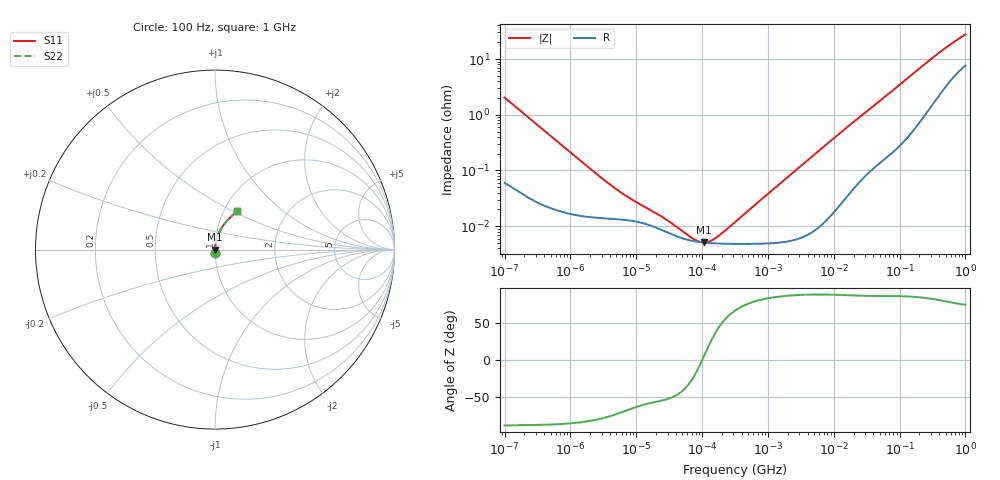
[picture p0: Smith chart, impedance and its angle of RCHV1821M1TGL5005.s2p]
! RCHV1821M1TGL5005  S-PARAMETER MODEL  (AEC-Q200 qualified)
! Model Generated by ELNA Corporation (http://www.ty-top.com)
! Version 1.0
! ELNA Control No. 240229
! Copyright (c) 2024 ELNA CO.,LTD. All Rights Reserved.
! Products Name : CONDUCTIVE POLYMER HYBRID ALUMINUM ELECTROLYTIC CAPACITORS
! Characteristics :
!  Capacitance  :  820uF  ,  Rated voltage  :  25V
!  Operating Temp. Range  :  -55 to +105 degC  ,  Endurance  :  5000hr at 105 degC
!  Dimension D  :  12.5mm  ,  Dimension L  :  13.5mm
! Frequency Range : 100Hz - 1GHz
! External Node Assignments :
!  1  o---| |---o  2
# MHz S RI R 50
!Freq[MHz].  S11 Real  S11 Imag  S21 Real  S21 Imag  S12 Real  S12 Imag  S22 Real  S22 Imag
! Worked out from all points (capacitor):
!   401 points, 100 Hz to 1 GHz, reference 50 ohm
!   read as one part in series: C = 781 uF near 108 Hz
!   lowest |Z| = 5.11 mohm at 106.5 kHz (marker M1)
!   series resonance near 101.1 kHz, so ESL is about 3.2 nH
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0.0001  0.00101 -0.0202  0.999 0.0202  0.999 0.0202  0.00101 -0.0202
0.000133  0.000726 -0.0153  0.9993 0.0153  0.9993 0.0153  0.000726 -0.0153
0.001488  0.000154 -0.00142  0.9998 0.00142  0.9998 0.00142  0.000154 -0.00142
0.00333  0.000139 -0.000645  0.9999 0.000645  0.9999 0.000645  0.000139 -0.000645
0.005855  0.000132 -0.000381  0.9999 0.000381  0.9999 0.000381  0.000132 -0.000381
0.00912  0.000123 -0.000261  0.9999 0.000261  0.9999 0.000261  0.000123 -0.000261
0.022131  8.97e-05 -0.000132  0.9999 0.000132  0.9999 0.000132  8.97e-05 -0.000132
0.037368  6.88e-05 -8.02e-05  0.9999 8.02e-05  0.9999 8.02e-05  6.88e-05 -8.02e-05
0.040504  6.63e-05 -7.3e-05  0.9999 7.3e-05  0.9999 7.3e-05  6.63e-05 -7.3e-05
0.043904  6.41e-05 -6.59e-05  0.9999 6.59e-05  0.9999 6.59e-05  6.41e-05 -6.59e-05
0.106537  5.1e-05 4e-06  0.9999 -4e-06  0.9999 -4e-06  5.1e-05 4e-06
0.248313  4.84e-05 7.88e-05  1 -7.88e-05  1 -7.88e-05  4.84e-05 7.88e-05
0.280221  4.83e-05 9.27e-05  1 -9.27e-05  1 -9.27e-05  4.83e-05 9.27e-05
0.316228  4.82e-05 0.000108  1 -0.000108  1 -0.000108  4.82e-05 0.000108
4.704354  8.12e-05 0.00179  0.9999 -0.00179  0.9999 -0.00179  8.12e-05 0.00179
16.4059  0.000393 0.00612  0.9996 -0.00612  0.9996 -0.00612  0.000393 0.00612
69.9842  0.00246 0.0242  0.9975 -0.0242  0.9975 -0.0242  0.00246 0.0242
169.8244  0.00879 0.0566  0.9912 -0.0566  0.9912 -0.0566  0.00879 0.0566
380.1894  0.034 0.1158  0.966 -0.1158  0.966 -0.1158  0.034 0.1158
641.9482  0.0741 0.1684  0.9259 -0.1684  0.9259 -0.1684  0.0741 0.1684
922.5714  0.114 0.2068  0.886 -0.2068  0.886 -0.2068  0.114 0.2068
1000  0.1239 0.2155  0.8761 -0.2155  0.8761 -0.2155  0.1239 0.2155
